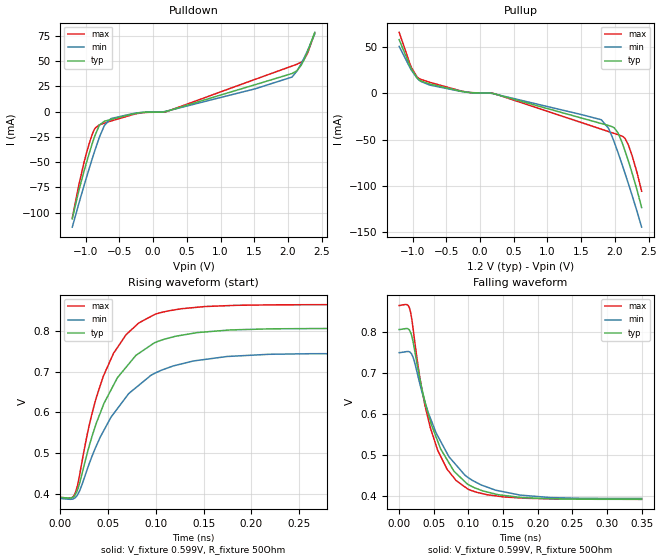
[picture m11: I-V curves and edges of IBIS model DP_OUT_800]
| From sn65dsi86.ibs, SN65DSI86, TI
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|   Model
[Model]   DP_OUT_800
Model_type   Output
Polarity   Non-Inverting
Vmeas = 0.6
Vref = 0.6
Cref = 1pF
Rref = 50
|   typ   min   max
C_comp   0.503pF   0.476pF   0.611pF
[Voltage Range]   1.2   1.14   1.26
[Temperature Range]   27   125   -40
[Pullup Reference]   1.2   1.14   1.26
[Pulldown Reference]   -0   -0   -0
[Power Clamp Reference]   1.2   1.14   1.26
[GND Clamp Reference]   -0   -0   -0
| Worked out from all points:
|   slope of the pulldown table from 0 to 0.18 V, typ, clamps not added: 377 ohm
|   slope of the pullup table from 0 to 0.18 V, typ, clamps not added: 458 ohm
|   falling waveform, V_fixture 0.599V, R_fixture 50Ohm: 20-80 % time 48.3ps typ, 58.4ps min, 40ps max; typ from 0.806 V to 0.391 V
|   rising waveform, V_fixture 0.599V, R_fixture 50Ohm: 20-80 % time 47.8ps typ, 57.4ps min, 39.6ps max; typ from 0.391 V to 0.806 V
[Pulldown]
|   Voltage   I(typ)   I(min)   I(max)
-1.2V     -106.2mA   -114.5mA   -105.3mA
-1.024V   -58.48mA   -72.9mA    -49.63mA
-904.8mV  -31.86mA   -46.82mA   -22.69mA
-789.6mV  -12.9mA    -24mA      -12.9mA
-721.2mV  -9.498mA   -13.47mA   -11.36mA
-624mV    -7.602mA   -6.816mA   -9.255mA
-199.2mV  -1.133mA   -965.2uA   -1.468mA
182.4mV   22.92uA    265.5uA    -243.5uA
2.058V    37.74mA    34.24mA    45.16mA
2.134V    40.69mA    40.41mA    47.03mA
2.238V    51.49mA    53.12mA    51.65mA
2.396V    78.6mA     76.88mA    77.89mA
[Pullup]
|   Voltage   I(typ)   I(min)   I(max)
-1.2V     58.3mA     51.01mA    66.22mA
-1.016V   26.24mA    24.96mA    27.87mA
-886.8mV  13.81mA    13.36mA    15.46mA
-249.6mV  1.931mA    1.797mA    2.203mA
182.4mV   67.48uA    -157.9uA   323.2uA
1.799V    -32.64mA   -28.55mA   -38.77mA
1.903V    -34.76mA   -37.67mA   -41.29mA
1.99V     -37.33mA   -52.69mA   -43.37mA
2.051V    -43.55mA   -65.1mA    -44.85mA
2.152V    -62.65mA   -86.97mA   -49mA
2.256V    -86.47mA   -110.8mA   -67.74mA
2.396V    -123.7mA   -145mA     -106mA
[Ramp]
R_load = 50
|   typ   min   max
dV/dt_r   0.248858/4.7752e-11   0.213339/5.73544e-11   0.284109/3.96296e-11
dV/dt_f   0.248858/4.83214e-11   0.21364/5.83987e-11   0.284109/3.99522e-11
[Falling Waveform]
V_fixture = 0.599V
V_fixture_min = 0.569V
V_fixture_max = 0.628V
R_fixture = 50Ohm
C_fixture = 0F
|   Time   V(typ)   V(min)   V(max)
0s        806.2mV    749.7mV    864.9mV
14.88ps   804.9mV    751.6mV    858.8mV
20.26ps   775.1mV    737.8mV    806.6mV
33.11ps   659.8mV    652.8mV    657mV
44.99ps   582.3mV    590.1mV    566.2mV
55.72ps   533mV      546.1mV    510.8mV
82.37ps   454.7mV    475mV      437.1mV
118.4ps   413.5mV    426.5mV    406mV
174.5ps   396.3mV    401.8mV    394.9mV
350ps     391.5mV    393.7mV    391.4mV
[Rising Waveform]
V_fixture = 0.599V
V_fixture_min = 0.569V
V_fixture_max = 0.628V
R_fixture = 50Ohm
C_fixture = 0F
|   Time   V(typ)   V(min)   V(max)
0s        391.5mV    388.7mV    391.4mV
14.88ps   394.8mV    389.4mV    397.3mV
20.26ps   425.7mV    407.2mV    445.5mV
33.11ps   539.6mV    491.2mV    595.6mV
44.99ps   617.2mV    552.9mV    688.2mV
55.72ps   666.7mV    596.5mV    744.8mV
82.37ps   745.2mV    666.9mV    819.9mV
118.4ps   785.6mV    714.2mV    851.3mV
174.5ps   801.9mV    737.3mV    862.1mV
350ps     806.2mV    744.2mV    864.9mV
